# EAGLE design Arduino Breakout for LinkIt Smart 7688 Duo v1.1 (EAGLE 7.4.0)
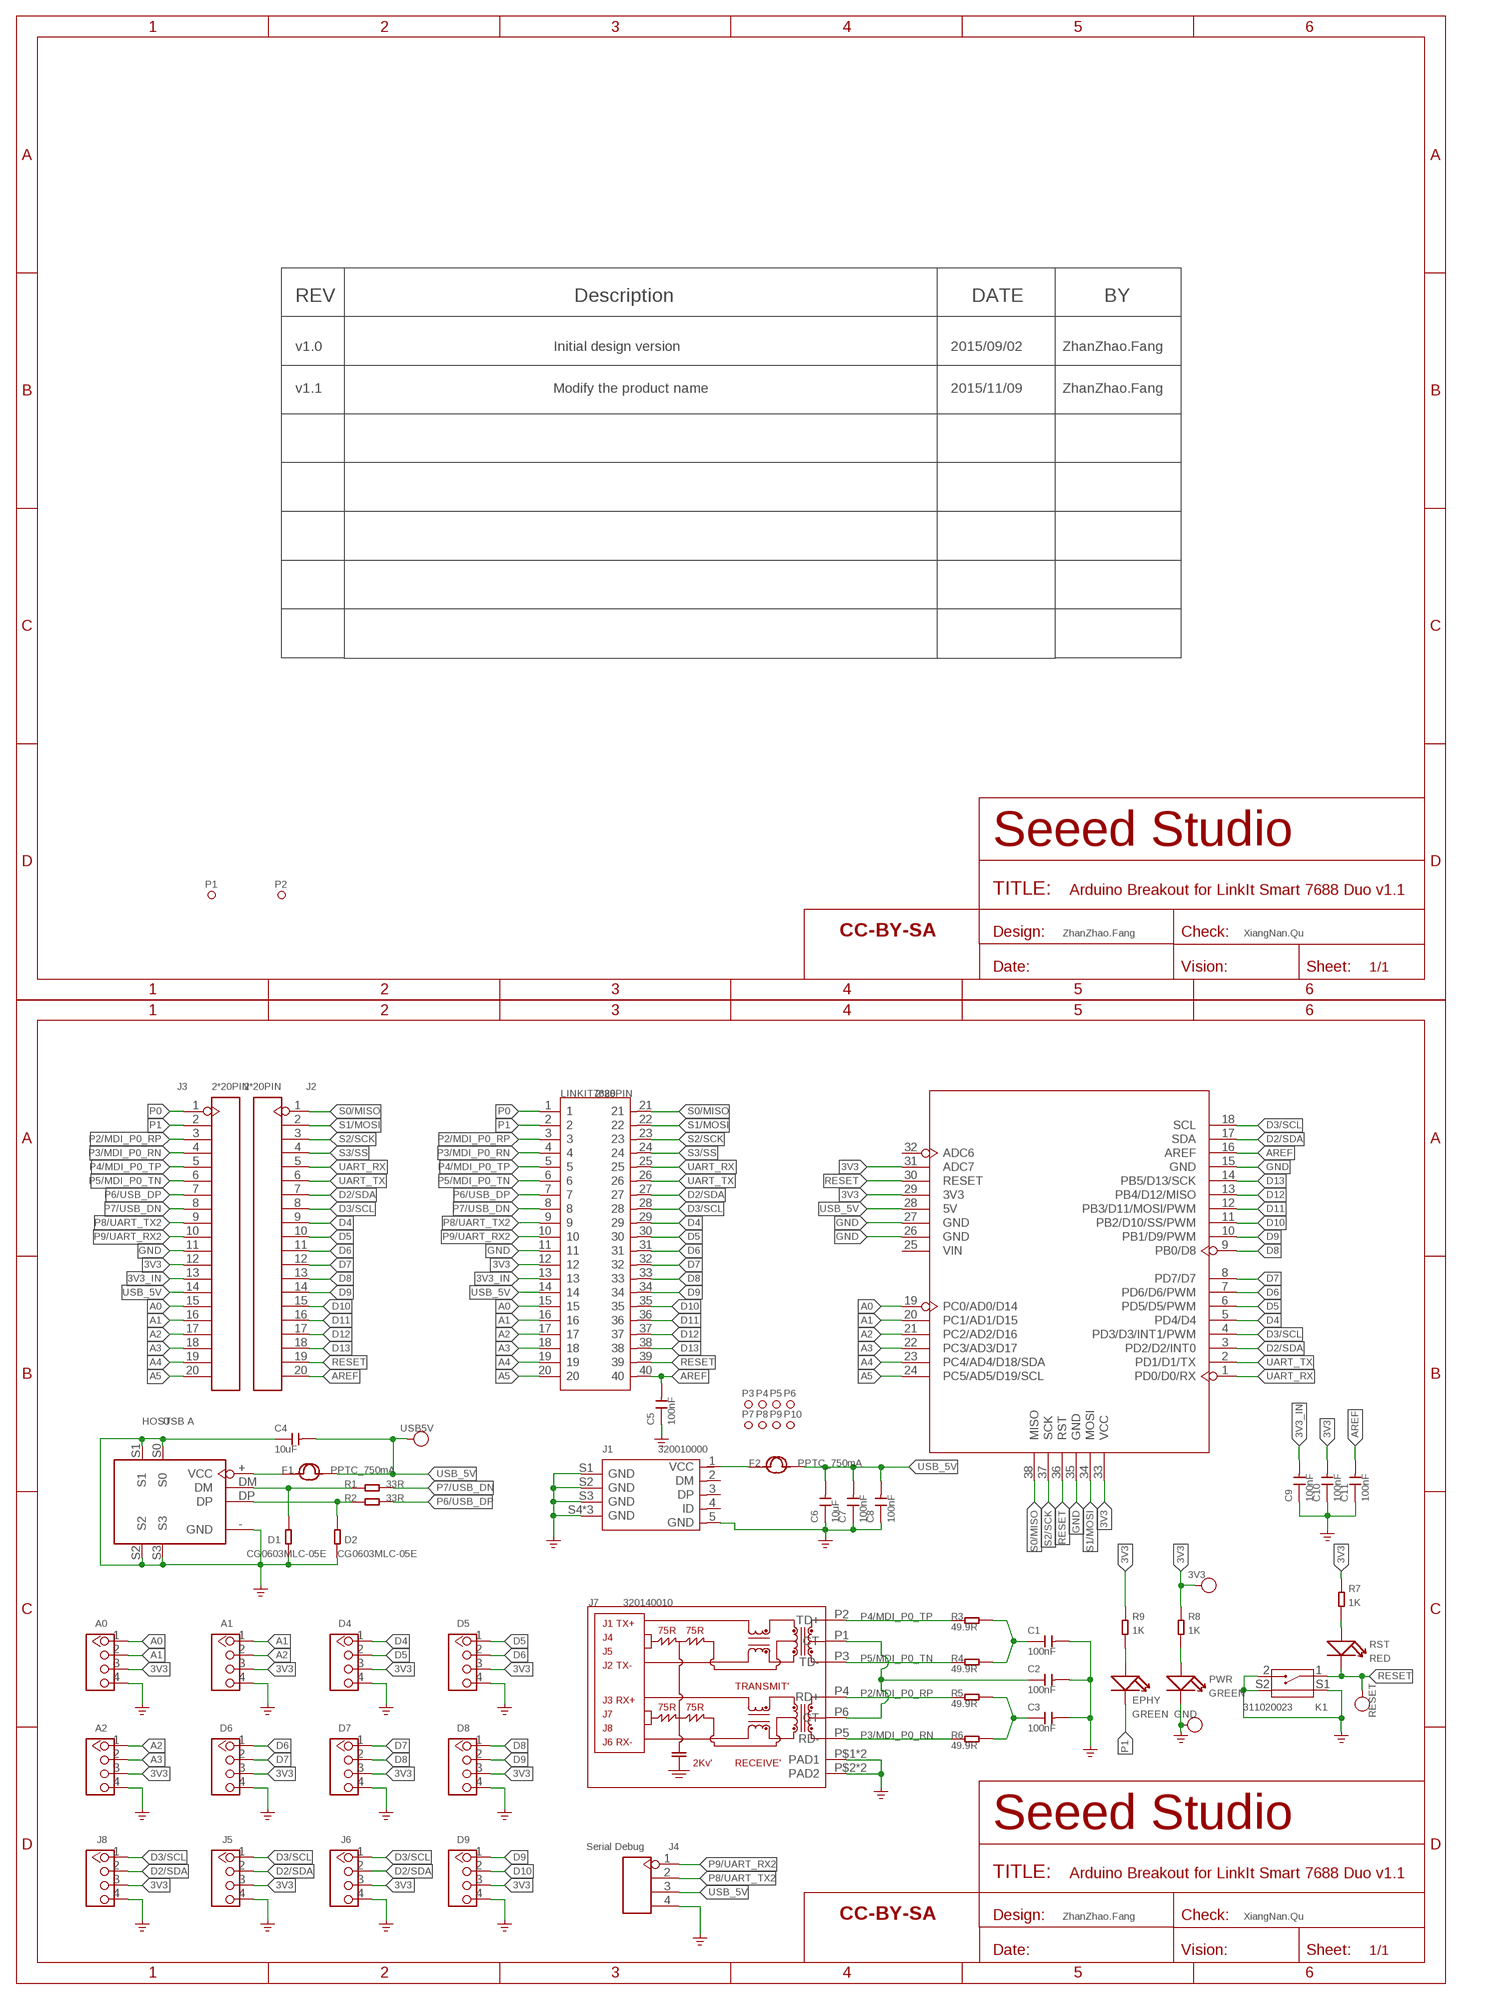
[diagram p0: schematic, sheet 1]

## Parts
3V3  DNP  TEST-POINT'4545'  [TP-D45MIL]
A0  320110033  GROVE-CONNECTOR-DIP-2.0  [HW4-2.0]
A1  320110033  GROVE-CONNECTOR-DIP-2.0  [HW4-2.0]
A2  320110033  GROVE-CONNECTOR-DIP-2.0  [HW4-2.0]
C1  100nF  CAP-0603  [C0603]
C2  100nF  CAP-0603  [C0603]
C3  100nF  CAP-0603  [C0603]
C4  10uF  CAP-0805  [C0805]
C5  100nF  CAP-0603  [C0603]
C6  10uF  CAP-0805  [C0805]
C7  100nF  CAP-0603  [C0603]
C8  100nF  CAP-0603  [C0603]
C9  100nF  CAP-0603  [C0603]
C10  100nF  CAP-0603  [C0603]
C11  100nF  CAP-0603  [C0603]
D1  CG0603MLC-05E  RES-0603  [R0603]
D2  CG0603MLC-05E  RES-0603  [R0603]
D4  320110033  GROVE-CONNECTOR-DIP-2.0  [HW4-2.0]
D5  320110033  GROVE-CONNECTOR-DIP-2.0  [HW4-2.0]
D6  320110033  GROVE-CONNECTOR-DIP-2.0  [HW4-2.0]
D7  320110033  GROVE-CONNECTOR-DIP-2.0  [HW4-2.0]
D8  320110033  GROVE-CONNECTOR-DIP-2.0  [HW4-2.0]
D9  320110033  GROVE-CONNECTOR-DIP-2.0  [HW4-2.0]
EPHY  GREEN  LED'0603'  [LED-0603]
F1  PPTC_750mA  FUSE'1206'  [F1206]
F2  PPTC_750mA  FUSE'1206'  [F1206]
FR1  DNP  SEEEDSTUDIO-OPEN-SCH-FRAME  [SEEEDSTUDIO-PCB-FRAME]
FR2  DNP  SEEEDSTUDIO-OPEN-SCH-FRAME  [SEEEDSTUDIO-PCB-FRAME]
GND  DNP  TEST-POINT'4545'  [TP-D45MIL]
HOST  USB A  USB4+4P-13.2X14.5  [USB4+4-90D-IN]
J1  320010000  MICRO-USB5+4P'5+4P'  [MICRO-USB5+4P-SMD-0.65-B]
J2  2*20PIN  HEADER-20P-2.54  [H20-2.54]
J3  2*20PIN  HEADER-20P-2.54  [H20-2.54]
J4  Serial Debug  HEADER-4P-90D  [H4-2.54-90D-MALE]
J5  320110033  GROVE-CONNECTOR-DIP-2.0  [HW4-2.0]
J6  320110033  GROVE-CONNECTOR-DIP-2.0  [HW4-2.0]
J7  320140010  RJ45-MJ6-BX11-RVS1T073  [RJ45-MJ6-BX11-RVS1T073]
J8  320110033  GROVE-CONNECTOR-DIP-2.0  [HW4-2.0]
K1  311020023  BUTTON-2+2P'TS-1188E'  [SW4-SMD-7.0X3.5X3.5MM-90D]
LINKIT7688  2*20PIN  LINKIT-7688-DUO  [HEADER-2X20P-2.54-65/35MIL]
P1  DNP  MARK-1.0'ANNULAR'  [ROUND-MARK-1.0]
P2  DNP  MARK-1.0'ANNULAR'  [ROUND-MARK-1.0]
P3  MARK-1.0'ANNULAR'  [ROUND-MARK-1.0]
P4  MARK-1.0'ANNULAR'  [ROUND-MARK-1.0]
P5  MARK-1.0'ANNULAR'  [ROUND-MARK-1.0]
P6  MARK-1.0'ANNULAR'  [ROUND-MARK-1.0]
P7  MARK-1.0'ANNULAR'  [ROUND-MARK-1.0]
P8  MARK-1.0'ANNULAR'  [ROUND-MARK-1.0]
P9  MARK-1.0'ANNULAR'  [ROUND-MARK-1.0]
P10  MARK-1.0'ANNULAR'  [ROUND-MARK-1.0]
PWR  GREEN  LED'0603'  [LED-0603]
R1  33R  RES-0603  [R0603]
R2  33R  RES-0603  [R0603]
R3  49.9R  RES-0603  [R0603]
R4  49.9R  RES-0603  [R0603]
R5  49.9R  RES-0603  [R0603]
R6  49.9R  RES-0603  [R0603]
R7  1K  RES-0603  [R0603]
R8  1K  RES-0603  [R0603]
R9  1K  RES-0603  [R0603]
RESET  DNP  TEST-POINT'4545'  [TP-D45MIL]
RST  RED  LED'0603'  [LED-0603]
U2  Shield  ARDUINO-38PWITH-SILK  [ARDUINO-DIM-WITH-SILK]
USB5V  DNP  TEST-POINT'4545'  [TP-D45MIL]

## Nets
3V3: 3V3.T A0.3 A1.3 A2.3 C10.2 D4.3 D5.3 D6.3 D7.3 D8.3 D9.3 J3.12 J5.3 J6.3 J8.3 LINKIT7688.12 R7.2 R8.2 R9.2 U2.29(3V3) U2.31(ADC7) U2.33(VCC)
3V3_IN: C9.2 J3.13 LINKIT7688.13
A0: A0.1 J3.15 LINKIT7688.15 U2.19(PC0/AD0/D14)
A1: A0.2 A1.1 J3.16 LINKIT7688.16 U2.20(PC1/AD1/D15)
A2: A1.2 A2.1 J3.17 LINKIT7688.17 U2.21(PC2/AD2/D16)
A3: A2.2 J3.18 LINKIT7688.18 U2.22(PC3/AD3/D17)
A4: J3.19 LINKIT7688.19 U2.23(PC4/AD4/D18/SDA)
A5: J3.20 LINKIT7688.20 U2.24(PC5/AD5/D19/SCL)
AREF: C5.2 C11.2 J2.20 LINKIT7688.40 U2.16(AREF)
D2/SDA: J2.7 J5.2 J6.2 J8.2 LINKIT7688.27 U2.3(PD2/D2/INT0) U2.17(SDA)
D3/SCL: J2.8 J5.1 J6.1 J8.1 LINKIT7688.28 U2.4(PD3/D3/INT1/PWM) U2.18(SCL)
D4: D4.1 J2.9 LINKIT7688.29 U2.5(PD4/D4)
D5: D4.2 D5.1 J2.10 LINKIT7688.30 U2.6(PD5/D5/PWM)
D6: D5.2 D6.1 J2.11 LINKIT7688.31 U2.7(PD6/D6/PWM)
D7: D6.2 D7.1 J2.12 LINKIT7688.32 U2.8(PD7/D7)
D8: D7.2 D8.1 J2.13 LINKIT7688.33 U2.9(PB0/D8)
D9: D8.2 D9.1 J2.14 LINKIT7688.34 U2.10(PB1/D9/PWM)
D10: D9.2 J2.15 LINKIT7688.35 U2.11(PB2/D10/SS/PWM)
D11: J2.16 LINKIT7688.36 U2.12(PB3/D11/MOSI/PWM)
D12: J2.17 LINKIT7688.37 U2.13(PB4/D12/MISO)
D13: J2.18 LINKIT7688.38 U2.14(PB5/D13/SCK)
GND: A0.4 A1.4 A2.4 C1.2 C2.2 C3.2 C4.1 C5.1 C6.1 C7.1 C8.1 C9.1 C10.1 C11.1 D1.1 D2.1 D4.4 D5.4 D6.4 D7.4 D8.4 D9.4 GND.T HOST.-(GND) HOST.S0 HOST.S1 HOST.S2 HOST.S3 J1.5(GND) J1.S1(GND) J1.S2(GND) J1.S3(GND) J1.S4(GND) J1.S5(GND) J1.S6(GND) J3.11 J4.4 J5.4 J6.4 J7.P$1(PAD1) J7.P$2(PAD2) J7.PAD1 J7.PAD2 J8.4 K1.2 K1.S1 K1.S2 LINKIT7688.11 PWR.- U2.15(GND) U2.26(GND) U2.27(GND) U2.35(GND) ; supply symbol labelled GND_POWER
N$1: PWR.+ R8.1
N$2: EPHY.+ R9.1
N$3: D2.2 HOST.DP R2.1
N$4: D1.2 HOST.DM R1.1
N$5: F1.1 HOST.+(VCC)
N$6: C2.1 J7.P1(CT) J7.P6(CT)
N$7: R7.1 RST.+
N$8: F2.1 J1.1(VCC)
N$10: C1.1 R3.2 R4.2
N$12: C3.1 R5.2 R6.2
P0: J3.1 LINKIT7688.1
P1: EPHY.- J3.2 LINKIT7688.2
P2/MDI_P0_RP: J3.3 J7.P4(RD+) LINKIT7688.3 R5.1
P3/MDI_P0_RN: J3.4 J7.P5(RD-) LINKIT7688.4 R6.1
P4/MDI_P0_TP: J3.5 J7.P2(TD+) LINKIT7688.5 R3.1
P5/MDI_P0_TN: J3.6 J7.P3(TD-) LINKIT7688.6 R4.1
P6/USB_DP: J3.7 LINKIT7688.7 R2.2
P7/USB_DN: J3.8 LINKIT7688.8 R1.2
P8/UART_TX2: J3.9 J4.2 LINKIT7688.9
P9/UART_RX2: J3.10 J4.1 LINKIT7688.10
RESET: J2.19 K1.1 LINKIT7688.39 RESET.T RST.- U2.30(RESET) U2.36(RST)
S0/MISO: J2.1 LINKIT7688.21 U2.38(MISO)
S1/MOSI: J2.2 LINKIT7688.22 U2.34(MOSI)
S2/SCK: J2.3 LINKIT7688.23 U2.37(SCK)
S3/SS: J2.4 LINKIT7688.24
UART_RX: J2.5 LINKIT7688.25 U2.1(PD0/D0/RX)
UART_TX: J2.6 LINKIT7688.26 U2.2(PD1/D1/TX)
USB_5V: C4.2 C6.2 C7.2 C8.2 F1.2 F2.2 J3.14 J4.3 LINKIT7688.14 U2.28(5V) USB5V.T
Unconnected: J1.2(DM) J1.3(DP) J1.4(ID) U2.25(VIN) U2.32(ADC6)

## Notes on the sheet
- REV | Description | DATE | BY
- v1.0 | Initial design version | 2015/09/02 | ZhanZhao.Fang
- v1.1 | Modify the product name | 2015/11/09 | ZhanZhao.Fang
- ZhanZhao.Fang | XiangNan.Qu
- ZhanZhao.Fang | XiangNan.Qu

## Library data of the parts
3V3 GND RESET USB5V = Discrete-new:TEST-POINT; PARTNO: DNP
A0 A1 A2 D4-D9 J5 J6 J8 = Connector-new:GROVE-CONNECTOR-DIP: 4P-2.0:320110033;4P-2.0-90D:320110034
C1-C11 = Discrete-new:CAP: Ceramic Capacitors
D1 D2 R1-R9 = Discrete-new:RES
EPHY PWR RST = Discrete-new:LED
F1 F2 = Discrete-new:FUSE
FR1 FR2 = moudle-new:SEEEDSTUDIO-OPEN-SCH-FRAME
HOST = Connector-new:USB4+4P: 320010017 USB-A-FEMALE
J1 = Connector-new:MICRO-USB5+4P: 5+4P-SMD-0.65-B:320010000;5+2P-SMD-0.65-AB:340032001
J2 J3 = Connector-new:HEADER-20P
J4 = Connector-new:HEADER-4P
J7 = Connector-new:RJ45-MJ6-BX11-RVS1T073: 320140010
K1 = Discrete-new:BUTTON-2+2P: SW4-SMD-4.5X3.8X1.8MM-90D:311020035;SW4-SMD-7.0X3.5X3.5MM-90D:311020023
LINKIT7688 = template:LINKIT-7688-DUO
P1-P10 = Discrete-new:MARK-1.0; PARTNO: DNP
U2 = moudle-new:ARDUINO-38P

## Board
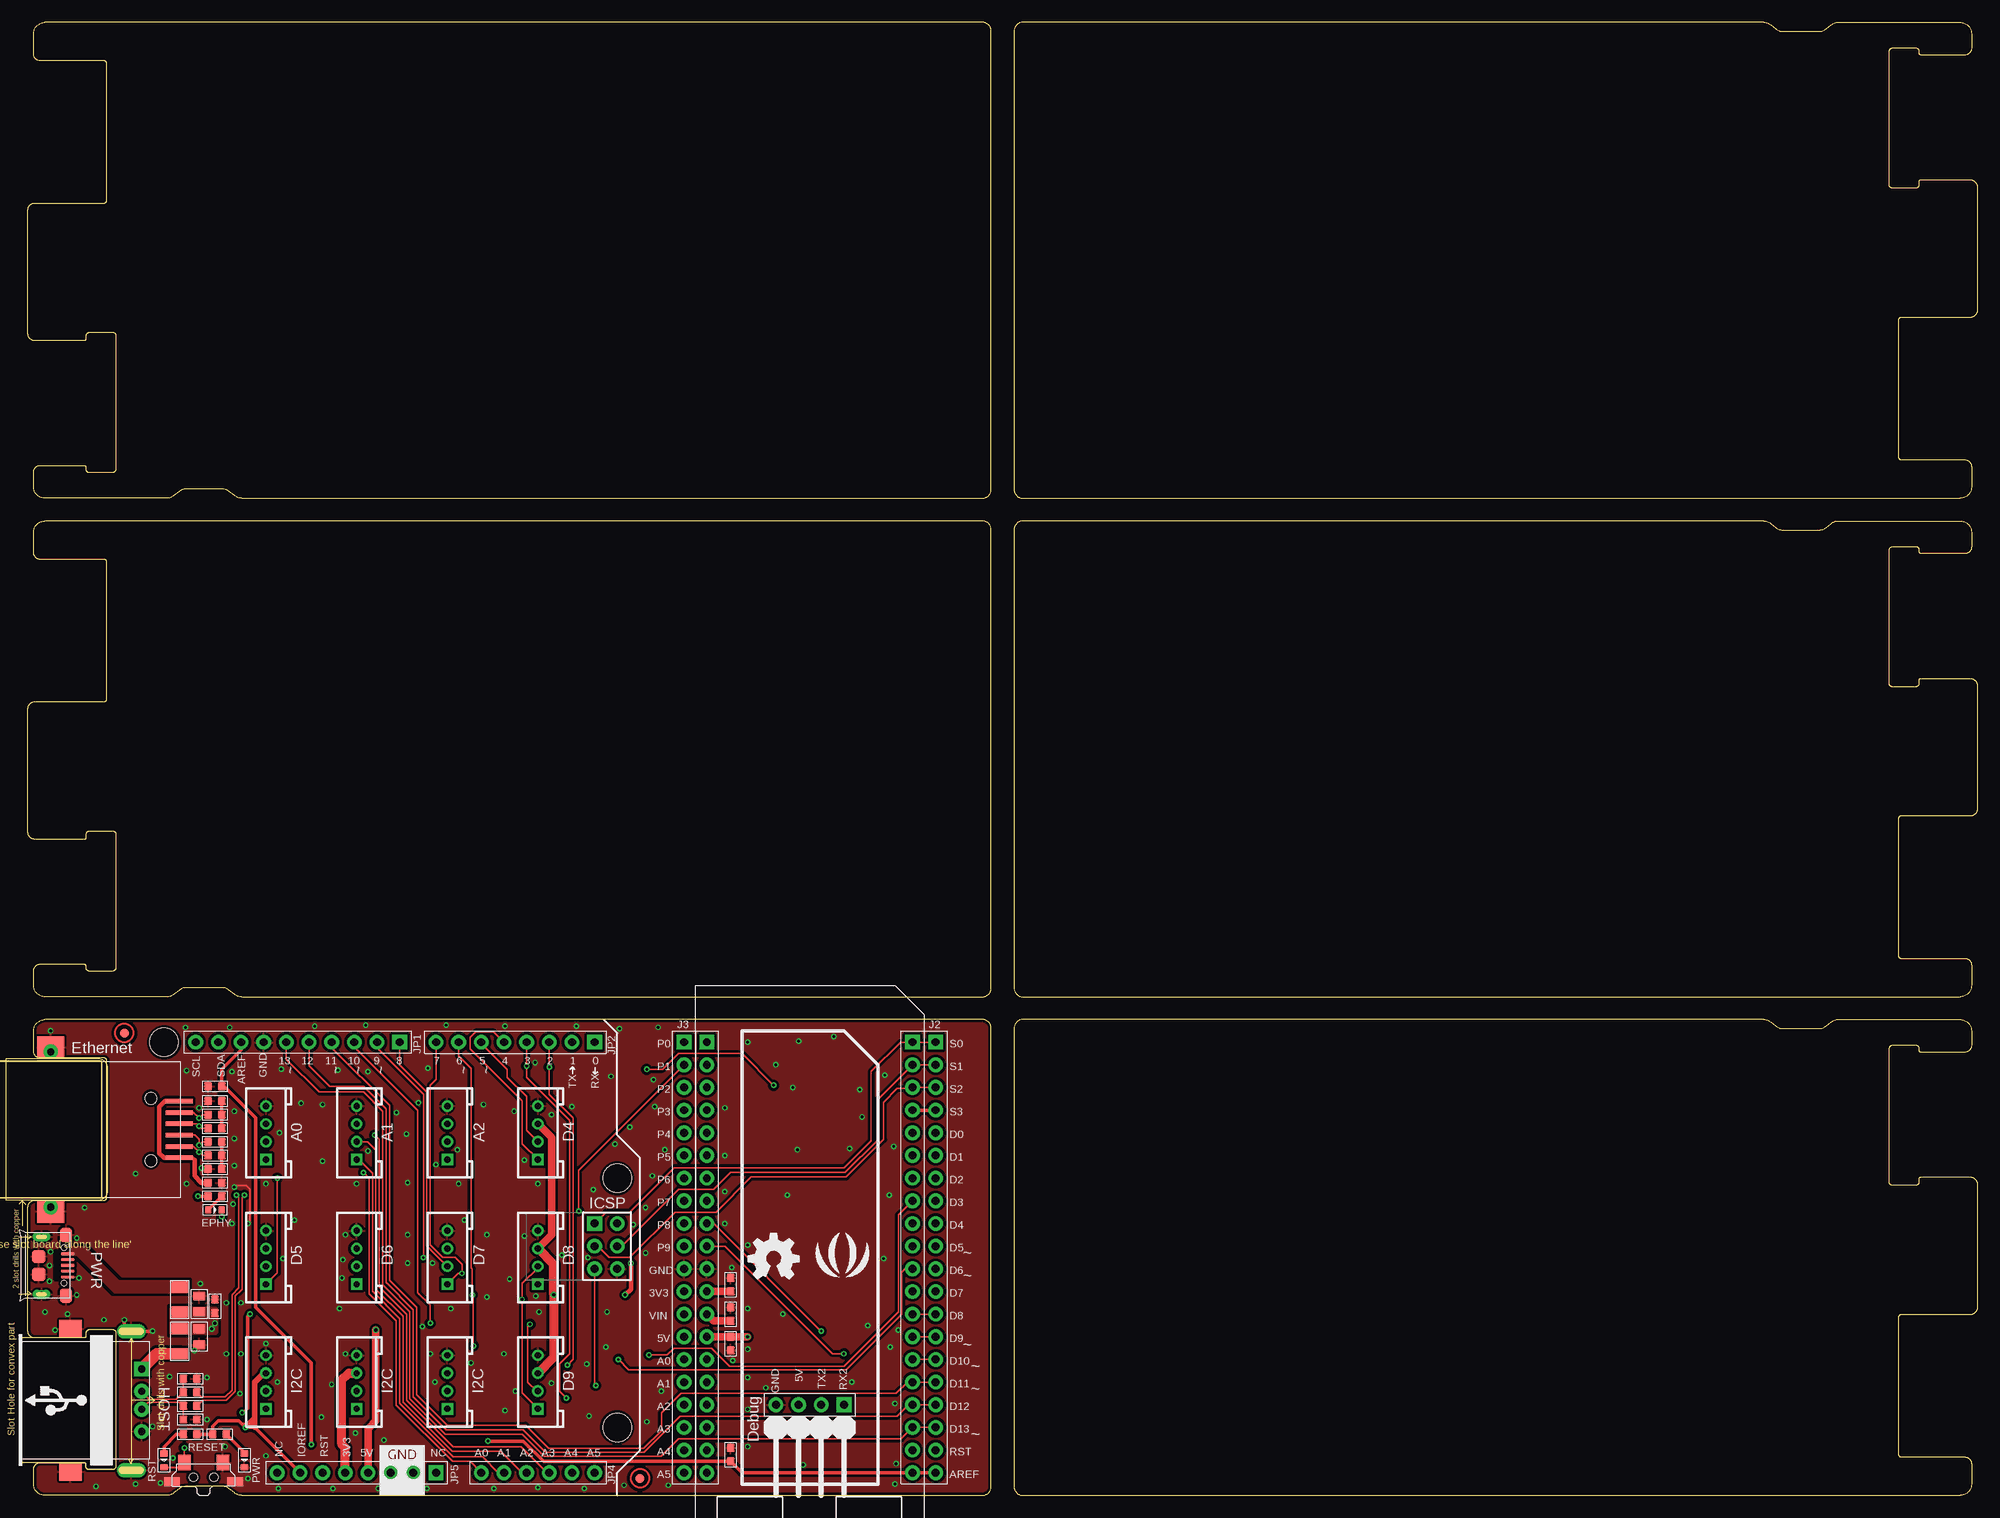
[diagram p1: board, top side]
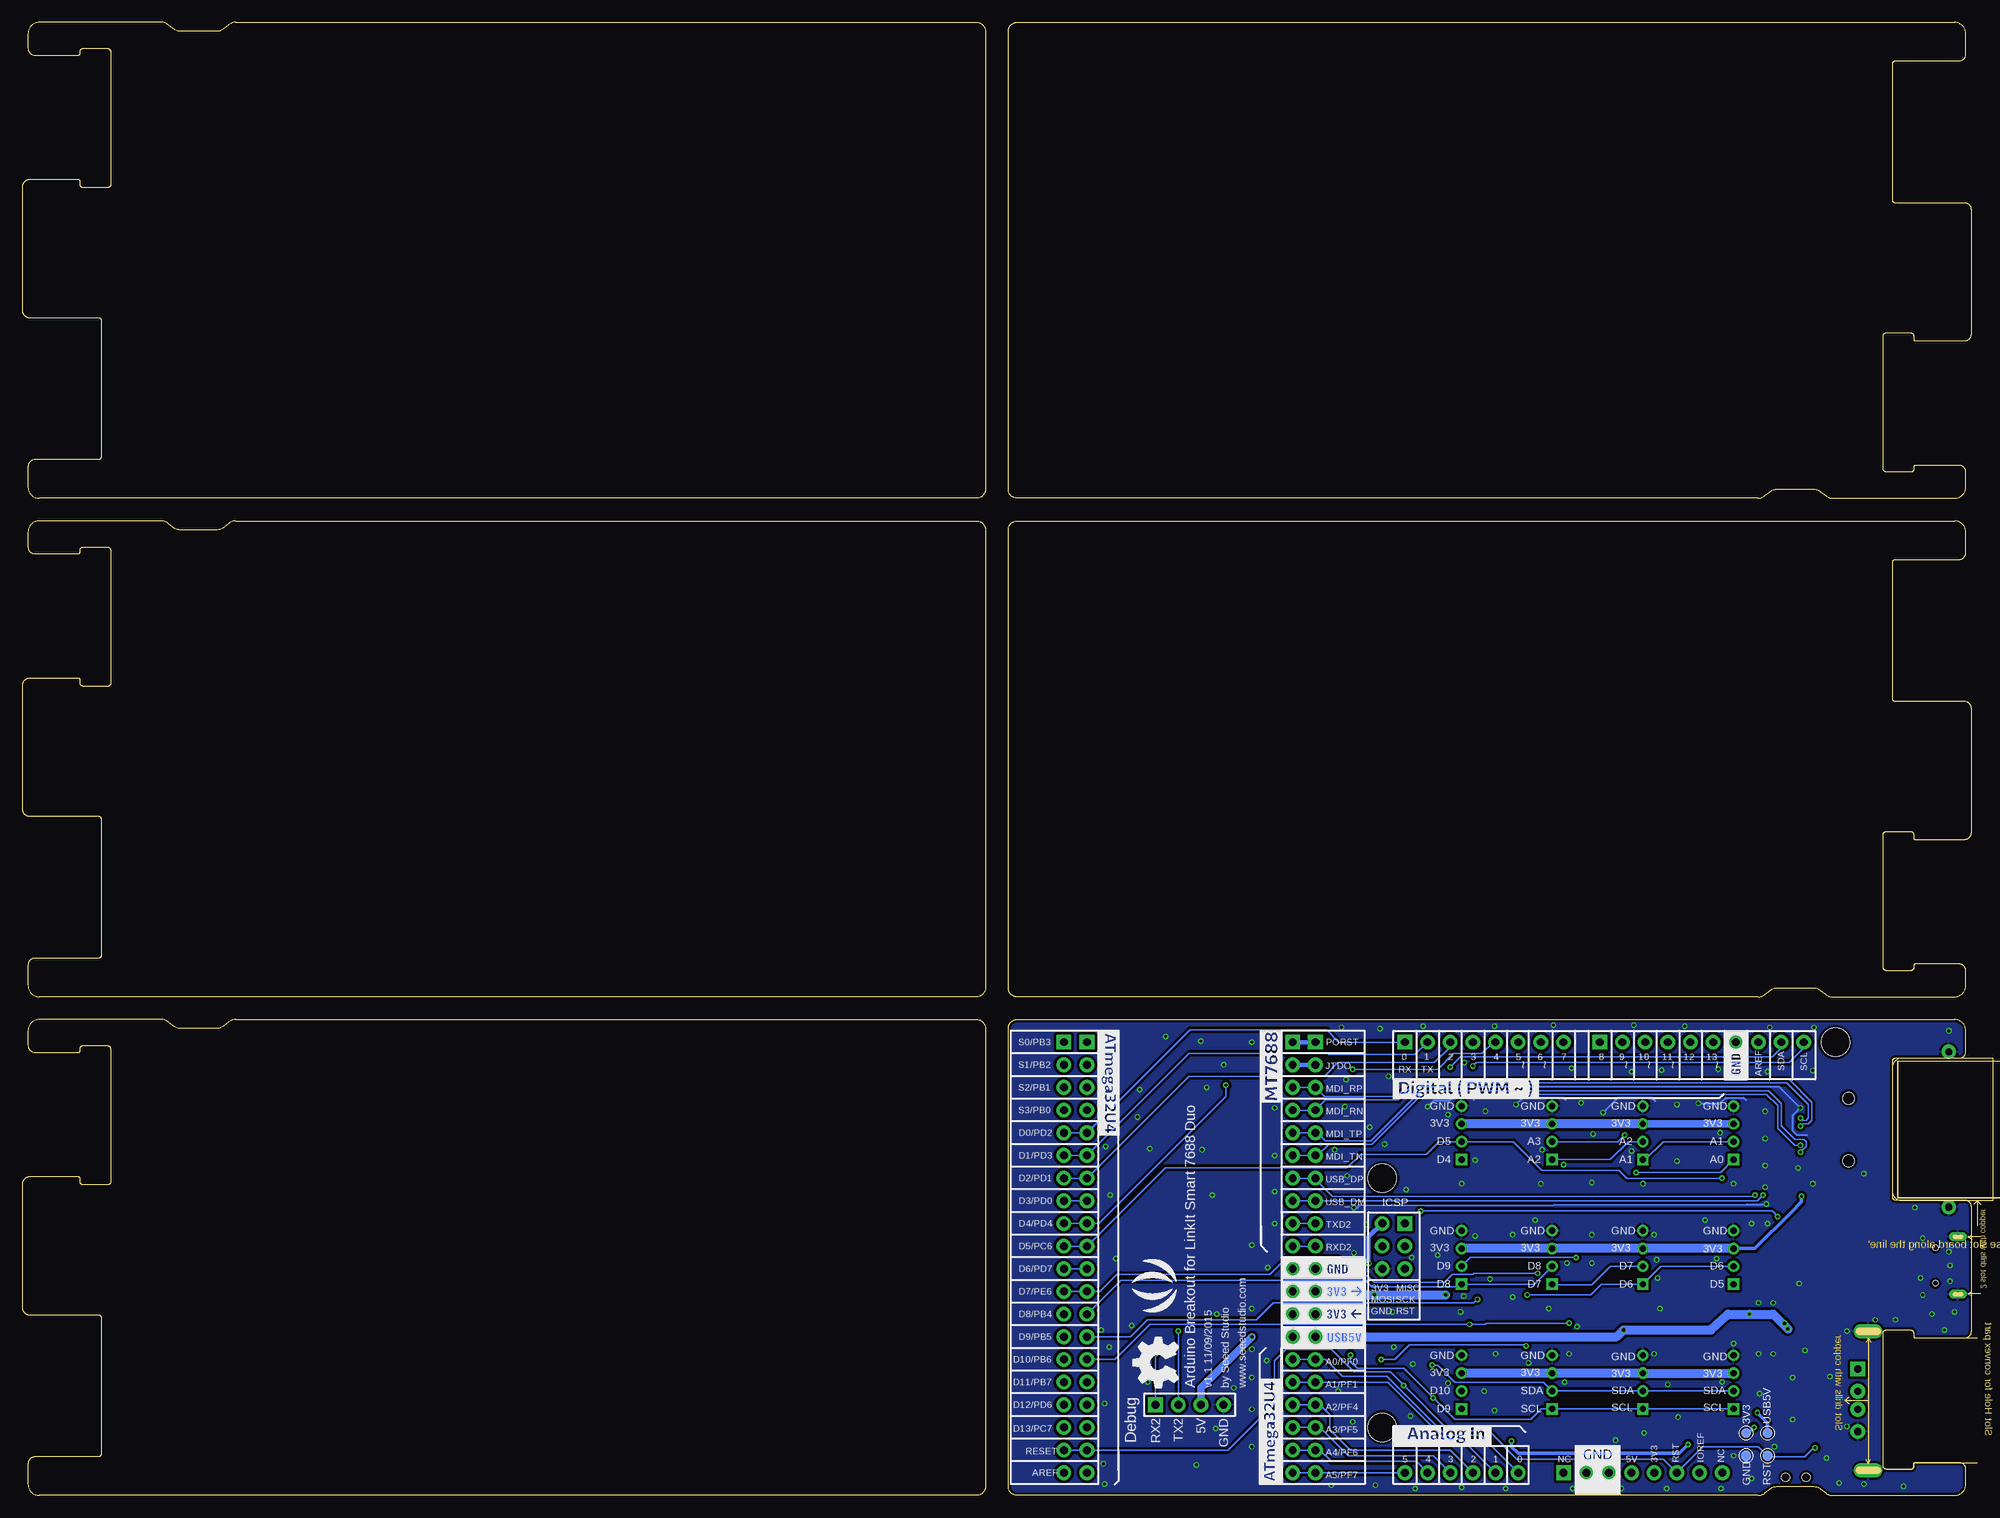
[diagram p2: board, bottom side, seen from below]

Size 219.07 x 165.1 mm. Coordinates in mm from the lower left corner, seen from the top.
Outline: 240 segments
Copper layers (1*16): Top 0.035mm / dielectric 1.5mm / Bottom 0.035mm
Design rules "SeeedStudio_2layer_DRU_no_angle_20140221 *": minimum track width 1mil, minimum drill 12mil, track to track 6mil, track to pad 6mil, pad to pad 6mil, via to via 6mil, smd to smd 0mil, copper to edge 10mil, drill to drill 10mil, minimum pad ring 10mil, minimum via ring 6mil, stop-mask expansion 2mil, vias tented up to drill 25mil, thermal gap 10mil
Holes 2 mm at 3.17,169.54 216.53,169.54 3.17,-4.45 216.53,-4.45

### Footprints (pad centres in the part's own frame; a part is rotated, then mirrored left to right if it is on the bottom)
TP-D45MIL = smd 1.143 x 1.143: T 0,0
HW4-2.0 = drill 0.7 pad 1.27 square: 1 -3,0 | drill 0.7 pad 1.27: 2 -1,0; 3 1,0; 4 3,0
C0603 = smd 0.889 x 0.889: 1 0,0.762; 2 0,-0.762
C0805 = smd 1.397 x 1.016: 1 0,0.889; 2 0,-0.889
R0603 = smd 0.889 x 0.889: 1 0,0.762; 2 0,-0.762
LED-0603 = smd 0.762 x 0.889: + -0.762,0; - 0.762,0
F1206 = smd 1.27 x 1.778: 1 -1.397,0; 2 1.397,0
USB4+4-90D-IN = drill 0.813 pad 1.651 square: + 0.85,-3.5 | drill 0.813 pad 1.651: - 0.85,3.5; DM 0.85,-1; DP 0.85,1 | smd 2.54 x 2.032: S0 8.83,8.001; S3 8.83,-8.001 | drill 0.7 pad 1.6 long: S1 2,7.874; S2 2,-7.747
MICRO-USB5+4P-SMD-0.65-B = smd 0.381 x 1.524: 1 -1.3,-0.25; 2 -0.65,-0.25; 3 0,-0.25; 4 0.65,-0.25; 5 1.3,-0.25 | smd 1.6 x 1.397: S1 -3.4,-0.427; S6 3.4,-0.427 | drill 0.508 pad 1.016 long: S2 -3.226,-3.175; S5 3.226,-3.175 | smd 1.5 x 1.5: S3 -1,-3.5; S4 1,-3.5 | hole 0.635: -2,-0.65; 2,-0.65
H20-2.54 = drill 0.889 pad 1.651 square: 1 0,-24.13 | drill 0.889 pad 1.651: 2 0,-21.59; 3 0,-19.05; 4 0,-16.51; 5 0,-13.97; 6 0,-11.43; 7 0,-8.89; 8 0,-6.35; 9 0,-3.81; 10 0,-1.27; 11 0,1.27; 12 0,3.81; 13 0,6.35; 14 0,8.89; 15 0,11.43; 16 0,13.97; 17 0,16.51; 18 0,19.05; 19 0,21.59; 20 0,24.13
H4-2.54-90D-MALE = drill 0.889 pad 1.651 square: 1 0,3.81 | drill 0.889 pad 1.651: 2 0,1.27; 3 0,-1.27; 4 0,-3.81
RJ45-MJ6-BX11-RVS1T073 = smd 0.5 x 3: P1 3.175,14.4; P2 1.905,14.4; P3 0.635,14.4; P4 -0.635,14.4; P5 -1.905,14.4; P6 -3.175,14.4 | smd 2.5 x 3: P$1 -9.2,0; P$2 9.2,0 | drill 0.8 pad 1.6: PAD1 -8.7,0; PAD2 8.7,0 | hole 1.35: -3.5,11.24; 3.5,11.24
SW4-SMD-7.0X3.5X3.5MM-90D = smd 1.397 x 1.778: 1 -2.159,1.651; 2 2.159,1.651 | smd 1.778 x 1.016: S1 -3.556,-0.508; S2 3.556,-0.508 | hole 0.95: -1.15,0; 1.15,0
HEADER-2X20P-2.54-65/35MIL = drill 0.889 pad 1.651 square: 1 0,24.13; 21 23.05,24.13 | drill 0.889 pad 1.651: 2 0,21.59; 3 0,19.05; 4 0,16.51; 5 0,13.97; 6 0,11.43; 7 0,8.89; 8 0,6.35; 9 0,3.81; 10 0,1.27; 11 0,-1.27; 12 0,-3.81; 13 0,-6.35; 14 0,-8.89; 15 0,-11.43; 16 0,-13.97; 17 0,-16.51; 18 0,-19.05; 19 0,-21.59; 20 0,-24.13; 22 23.05,21.59; 23 23.05,19.05; 24 23.05,16.51; 25 23.05,13.97; 26 23.05,11.43; 27 23.05,8.89; 28 23.05,6.35; 29 23.05,3.81; 30 23.05,1.27; 31 23.05,-1.27; 32 23.05,-3.81; 33 23.05,-6.35; 34 23.05,-8.89; 35 23.05,-11.43; 36 23.05,-13.97; 37 23.05,-16.51; 38 23.05,-19.05; 39 23.05,-21.59; 40 23.05,-24.13
ROUND-MARK-1.0 = smd 1.016 x 1.016: P$1 0,0
ARDUINO-DIM-WITH-SILK = drill 0.889 pad 1.651 square: 1 63.5,50.8; 9 41.656,50.8; 25 45.72,2.54; 38 63.5,30.48 | drill 0.889 pad 1.651: 2 60.96,50.8; 3 58.42,50.8; 4 55.88,50.8; 5 53.34,50.8; 6 50.8,50.8; 7 48.26,50.8; 8 45.72,50.8; 10 39.116,50.8; 11 36.576,50.8; 12 34.036,50.8; 13 31.496,50.8; 14 28.956,50.8; 15 26.416,50.8; 16 23.876,50.8; 17 21.336,50.8; 18 18.796,50.8; 19 50.8,2.54; 20 53.34,2.54; 21 55.88,2.54; 22 58.42,2.54; 23 60.96,2.54; 24 63.5,2.54; 26 43.18,2.54; 27 40.64,2.54; 28 38.1,2.54; 29 35.56,2.54; 30 33.02,2.54; 31 30.48,2.54; 32 27.94,2.54; 33 66.04,30.48; 34 66.04,27.94; 35 66.04,25.4; 36 63.5,25.4; 37 63.5,27.94 | hole 3.2: 15.24,50.8; 66.04,35.56; 66.04,7.62

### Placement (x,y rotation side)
3V3  25.91,6.99 0 bottom
A0  27.3,40.64 90 top
A1  37.46,40.64 90 top
A2  47.62,40.64 90 top
C1  21.59,36.58 270 top
C2  21.59,35.05 90 top
C3  21.59,44.2 270 top
C4  19.81,17.78 180 top
C5  21.59,45.85 90 top
C6  19.81,21.46 0 top
C7  21.59,21.21 0 top
C8  79.38,17.02 180 top
C9  79.38,20.32 0 top
C10  79.38,23.62 0 top
C11  79.38,4.57 0 top
D1  18.8,13.08 270 top
D2  18.8,8.51 270 top
D4  57.78,40.64 90 top
D5  27.3,26.67 90 top
D6  37.46,26.67 90 top
D7  47.62,26.67 90 top
D8  57.78,26.67 90 top
D9  57.78,12.7 90 top
EPHY  21.59,32 0 top
F1  17.65,17.27 90 top
F2  17.65,21.97 270 top
FR1  not placed on the board
FR2  not placed on the board
GND  25.91,4.45 0 bottom
HOST  14.22,10.67 180 top
J1  5.33,25.78 270 top
J2  102.36,26.67 180 top
J3  74.17,26.67 180 top
J4  88.27,10.16 270 top
J5  37.46,12.7 90 top
J6  47.62,12.7 90 top
J7  3.17,41.02 270 top
J8  27.3,12.7 90 top
K1  20.32,2.03 0 top
LINKIT7688  76.71,26.67 0 top
P1  69.22,1.91 0 top
P2  11.43,51.82 0 top
P3  not placed on the board
P4  not placed on the board
P5  not placed on the board
P6  not placed on the board
P7  not placed on the board
P8  not placed on the board
P9  not placed on the board
P10  not placed on the board
PWR  24.89,3.94 270 top
R1  18.8,11.56 90 top
R2  18.8,10.03 90 top
R3  21.59,38.1 90 top
R4  21.59,39.62 90 top
R5  21.59,41.15 90 top
R6  21.59,42.67 90 top
R7  18.8,6.86 90 top
R8  22.1,6.86 270 top
R9  21.59,33.53 270 top
RESET  23.49,4.45 0 bottom
RST  15.88,3.94 270 top
U2  0.63,0 0 top
U$20  [OSHW_FILLX200_NOTEXT]  89.54,12.06 90 bottom
U$21  [SEEED-SILK-280*268MIL]  91.44,23.5 90 bottom
U$22  [OSHW_FILLX200_NOTEXT]  81.36,24.28 0 top
U$23  [SEEED-SILK-280*268MIL]  91.9,26.16 0 top
USB5V  23.49,6.99 0 bottom

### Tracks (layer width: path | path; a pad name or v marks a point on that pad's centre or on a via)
3V3  (via drill 0.3, 0.36, 0.38)
  Top 0.406: 24.64,8 24.26,8.38 21.97,8.38 21.34,7.75 R8.2 R7.2 | 24.64,8 v25.02,7.62 26.03,7.62 U2.31 | 24.64,8 25.53,8 | R9.2 v19.69,33.53
  Top 0.508: v67.56,22.48 68.2,23.11 v68.2,26
  Top 0.61: J8.3 27.03,13.7 26.03,12.7 26.03,8.64 | 26.03,8.64 25.65,8.26 | 25.65,8.26 v25.02,7.62 | 25.65,8.26 25.65,7.75 | 26.03,7.62 26.03,8.64
  Top 0.813: D4.3 59.31,40.12 59.31,29.19 D8.3 | C10.2 LINKIT7688.12
  Top 1.016: U2.29 36.2,5.33 35.81,5.71 35.81,12.94 36.58,13.7 J5.3 | D8.3 59.56,25.89 v59.56,22.48 59.56,15.48 D9.3
  Bottom 0.406: 3V3.T 25.65,6.99 v25.02,7.62 | D5.3 24.91,27.67 20.89,31.69 20.83,31.75 19.69,32.89 v19.69,33.53
  Bottom 0.508: U2.33 68.2,28.96 v68.2,26
  Bottom 0.813: A0.3 A1.3
  Bottom 1.016: D9.3 J6.3 J5.3 J8.3 | LINKIT7688.12 J3.12 69.09,22.86 68.71,22.48 v67.56,22.48 v59.56,22.48 | D5.3 D6.3 D7.3 D8.3 | A1.3 A2.3 D4.3
3V3_IN
  Top 0.813: C9.2 77.47,19.56 LINKIT7688.13
  Bottom 0.813: J3.13 LINKIT7688.13
A0  (via drill 0.3)
  Top 0.152: U2.19 50.16,3.81 48.23,3.81 41.91,10.13 41.91,19.56 38.86,22.61 38.86,35.56 v38.23,36.2
  Bottom 0.152: LINKIT7688.15 J3.15 73.03,15.24 71.12,13.34 66.17,13.34 59.56,6.73 55.63,6.73 U2.19 | v38.23,36.2 28.75,36.2 A0.1
A1
  Top 0.152: U2.20 53.34,2.54 51.56,4.32 48.28,4.32 42.29,10.31 42.29,19.81 39.24,22.86 39.24,36.07 37.67,37.64 A1.1
  Bottom 0.152: LINKIT7688.16 J3.16 66.04,12.7 59.69,6.35 57.78,6.35 U2.20 | A1.1 37.16,37.64 35.18,39.62 27.32,39.62 A0.2
A2
  Top 0.152: U2.21 56.01,2.54 53.59,4.95 48.19,4.95 42.67,10.47 42.67,20.07 39.62,23.11 39.62,38.73 38.72,39.64 A1.2
  Bottom 0.152: LINKIT7688.17 J3.17 73.66,10.16 72.52,9.02 72.52,7.37 70.23,5.08 59.05,5.08 U2.21 | A2.1 41.1,37.64 39.1,39.64 A1.2
A3  (via drill 0.3)
  Top 0.152: U2.22 58.8,2.54 55.88,5.46 48.28,5.46 43.05,10.69 43.05,20.32 40,23.37 40,39.88 v39.5,40.39
  Bottom 0.152: LINKIT7688.18 J3.18 73.66,7.62 70.48,4.45 60.96,4.45 U2.22 | A2.2 40.24,39.64 v39.5,40.39
A4
  Bottom 0.152: LINKIT7688.19 J3.19 73.66,5.08 72.39,3.81 62.86,3.81 U2.23
A5
  Bottom 0.152: LINKIT7688.20 J3.20 U2.24
AREF  (via drill 0.3)
  Top 0.406: U2.16 24.51,49.91 22.35,47.75 C5.2 22.61,45.85 26.16,42.29 26.16,21.08 32.38,14.86 v32.38,5.71 | J2.20 LINKIT7688.40 80.65,2.54 C11.2 58.42,3.81 56.13,6.1 v52.2,6.1
  Bottom 0.406: v52.2,6.1 52.2,5.46 51.43,4.7 33.4,4.7 v32.38,5.71
D2/SDA  (via drill 0.3)
  Top 0.152: U2.3 v59.05,48.01 59.05,44.96 61.72,42.29 61.72,15.24 v61.09,14.61
  Bottom 0.152: J2.7 LINKIT7688.27 88.33,46.99 73.15,46.99 71.63,48.51 60.83,48.51 59.05,50.29 U2.3 | U2.17 21.97,50.16 22.99,49.15 57.91,49.15 v59.05,48.01 | v61.09,14.61 60.45,14.61 58.55,12.7 48.62,12.7 J6.2 J5.2 J8.2
D3/SCL  (via drill 0.3)
  Top 0.152: U2.4 v56.52,48.13 56.52,46.86 61.34,42.04 61.34,15.88 60.2,14.73 60.2,11.68 v60.96,10.92 | LINKIT7688.28 98.17,31.43 98.17,20.57 92.08,14.48 79.25,14.48 77.22,16.51 73.03,16.51 72.26,15.75 v70.23,15.75
  Bottom 0.152: U2.18 19.43,50.16 21.08,48.51 56.13,48.51 v56.52,48.13 | LINKIT7688.28 J2.8 | v70.23,15.75 70.23,14.99 69.47,14.22 64.26,14.22 v60.96,10.92 58.55,8.51 50.04,8.51 48.85,9.7 J6.1 J5.1 J8.1
D4  (via drill 0.3)
  Top 0.152: U2.5 52.83,51.94 50.8,51.94 50.16,51.31 50.16,50.04 56.01,44.2 56.01,39.42 D4.1 | v69.98,47.75 71.76,47.75 73.53,49.53 80.65,49.53 v84.2,45.97
  Bottom 0.152: J2.9 LINKIT7688.29 98.43,30.48 84.2,44.7 v84.2,45.97 | v69.98,47.75 60.45,47.75 58.67,49.53 55.5,49.53 54.23,50.8 U2.5
D5  (via drill 0.3)
  Top 0.152: U2.6 51.43,50.67 54.36,47.75 54.36,46.86 56.52,44.7 56.52,40.91 D4.2 | v28.58,35.56 28.58,24.94 D5.1
  Bottom 0.152: J2.10 LINKIT7688.30 91,36.7 70.61,36.7 69.09,38.23 61.72,38.23 60.32,39.62 57.8,39.62 D4.2 51.96,39.64 48.77,36.45 40.13,36.45 39.24,35.56 v28.58,35.56
D6  (via drill 0.3)
  Top 0.152: U2.7 48.89,49.28 50.29,47.88 50.29,25.53 50.42,25.4 v50.42,22.48 50.55,22.35 v50.55,16.76 | LINKIT7688.31 98.93,25.4 98.55,25.02 98.55,20.32 92.33,14.1 67.95,14.1 v66.8,15.24
  Bottom 0.152: LINKIT7688.31 J2.11 | D5.2 35.46,25.67 D6.1 42.12,23.67 43.31,22.48 v50.42,22.48 | v66.8,15.24 65.28,15.24 63.63,16.89 50.67,16.89 v50.55,16.76
D7  (via drill 0.3)
  Top 0.152: U2.8 46.35,46.61 45.72,45.97 45.72,28.07 47.12,26.67 48.51,26.67 49.28,25.91 v49.28,24.89 48.85,24.89 D7.1
  Bottom 0.152: J2.12 LINKIT7688.32 98.3,22.86 96.39,24.77 79.25,24.77 77.34,26.67 71.63,26.67 69.6,24.64 68.33,24.64 67.56,23.88 59.69,23.88 58.8,24.77 56.52,24.77 56.39,24.89 v49.28,24.89 | D6.2 41.13,25.67 43.18,23.62 47.58,23.62 D7.1
D8
  Top 0.152: J2.13 LINKIT7688.33 | D7.2 45.34,27.96 45.34,45.21 42.29,48.26 U2.9
  Bottom 0.152: LINKIT7688.33 95.95,24.13 68.58,24.13 67.82,23.37 58.09,23.37 D8.1 49.62,23.67 D7.2 47.77,25.53
D9  (via drill 0.3)
  Top 0.152: U2.10 39.75,50.16 44.96,44.96 v44.96,26.67 | J2.14 LINKIT7688.34 | D9.1 56.01,11.48 v56.01,21.97 56.01,23.75 57.78,25.53 D8.2
  Bottom 0.152: v56.01,21.97 56.39,21.59 78.87,21.59 80.77,19.68 92.96,19.68 94.87,17.78 LINKIT7688.34 | v44.96,26.67 56.78,26.67 D8.2
D10  (via drill 0.3)
  Top 0.152: U2.11 37.21,50.29 44.32,43.18 44.32,22.73 45.72,21.34 v45.72,19.3 | LINKIT7688.35 J2.15 | D9.2 57.64,11.7 56.64,12.7 56.64,18.92 v56.9,19.18
  Bottom 0.152: v45.72,19.3 54.99,19.3 55.12,19.18 v56.9,19.18 92.71,19.18 96.65,15.24 LINKIT7688.35
D11
  Top 0.152: J2.16 LINKIT7688.36 99.19,12.7 97.92,11.43 73.81,11.43 71.63,9.24 71.63,7.24 69.65,5.26 59,5.26 56.39,7.87 47.62,7.87 44.2,11.3 44.2,21.08 41.15,24.13 41.15,43.69 34.67,50.16 U2.12
D12
  Top 0.152: U2.13 32.13,48.13 34.42,45.85 38.23,45.85 40.77,43.31 40.77,23.88 43.81,20.83 43.81,11.05 47.5,7.37 56.13,7.37 58.64,4.86 69.7,4.86 73.73,8.89 98.04,8.89 99.31,10.16 LINKIT7688.37 J2.17
D13
  Top 0.152: U2.14 29.59,48.9 33.27,45.21 38.23,45.21 40.39,43.05 40.39,23.62 43.43,20.57 43.43,10.83 47.41,6.86 56.01,6.86 58.47,4.4 71.58,4.4 73.53,6.35 98.49,6.35 LINKIT7688.38 J2.18
GND  (via drill 0.3)
  Top 0.203: v25.27,30.48 25.53,30.73 25.53,34.29 25.15,34.67 23.88,34.67 v23.75,34.54
  Top 0.406: v11.43,19.68 11.43,19.18 12.19,18.41 v14.61,18.41
  Top 0.61: C1.2 20.19,36.58 v20.07,36.7
  Bottom 0.203: v69.85,32.26 69.47,32.26 69.22,32.51 25.78,32.64 v23.62,32.64 | 63.75,44.58 62.55,45.78 22.16,45.78 v19.81,43.43 20.7,42.55 20.7,40.89 20.19,40.39 19.05,40.39 | 56.39,44.32 56.64,44.58 58.8,44.58 59.18,44.2 60.96,44.2 v61.59,43.56 | 46.1,44.32 46.35,44.58 50.93,44.58 v51.69,43.81 | 36.07,44.2 36.45,44.58 40.26,44.58 v41.91,42.93 | v31.24,43.94 28.83,43.94 28.19,44.58 26.16,44.58 25.91,44.32
  other vias: 24.38,11.43 20.7,13.21 19.3,16.26 16.51,13.34 14.61,7.75 16.89,4.19 22.73,5.46 25.27,1.91 27.3,4.45 12.7,1.27 15.49,1.4 8.25,1.02 6.98,32.26 9.14,19.68 23.75,36.96 12.7,36.07 18.41,34.92 18.41,47.62 3.17,52.07 23.49,47.5 29.02,47.78 33.66,43.81 35.36,47.65 38.73,47.5 23.75,43.05 23.75,40.01 28.83,40.64 33.66,37.47 27.3,34.92 37.46,34.92 30.48,30.86 36.2,29.21 35.81,24.38 52.07,22.23 43.18,29.21 43.18,35.05 56.26,29.08 49.53,30.86 48.89,34.92 57.78,34.92 54.61,24.26 44.83,18.92 45.72,15.88 46.23,12.7 53.98,15.88 50.29,14.86 54.1,9.53 40.51,6.19 37.34,6.99 33.53,8.76 28.7,0.76 34.8,0.76 39.88,0.76 45.34,0.76 52.83,0.76 57.78,0.89 62.99,0.76 63.52,8.89 71.63,11.68 69.98,8.26 27.3,17.02 65.41,16.64 69.85,27.18 70.61,35.81 55.12,43.05 59.31,42.67 70.87,43.56 68.07,41.27 64.01,34.29 45.47,47.88 44.38,44 43.05,40.51 52.07,29.21 68.45,30.35 65.98,46.96 70.74,46.61 66.93,52.32 71.25,52.45 62.1,52.58 54.1,52.58 47.5,52.7 38.48,52.7 32.77,52.58 23.24,52.45 18.29,52.45 78.74,43.43 86.87,38.73 78.74,38.1 86.36,45.72 84.45,48.26 81.28,50.8 87,50.93 90.93,51.44 96.65,47.12 93.85,45.47 92.71,38.86 97.66,39.12 94.11,42.42 97.16,33.66 85.73,33.66 78.74,30.48 81.28,28.07 96.52,26.54 94.74,19.05 81.28,20.95 81.28,13.21 85.22,20.32 92.96,12.7 97.28,16.64 98.17,18.54 97.79,10.29 83.31,12.06 81.28,16.38 81.28,9.65 79.63,15.11 85.34,7.49 97.92,3.56 87.5,3.43 81.28,5.46 67.44,1.14 72.39,1.14 97.79,1.27 43.18,26.04 45.97,26.04 57.47,48.53 66.42,39.37 72.01,38.73 36.2,15.88 34.67,12.45 28.58,12.7 38.73,38.61 48.77,38.73 56.26,37.59 35.94,26.42 29.21,26.54 57.53,22.35 55.24,11.68 60.45,26.92 59.31,12.57 63.25,14.73 63.37,26.67 79.5,25.53 24.51,15.88 22.86,15.88 24.51,21.59 22.86,21.59 23.49,30.48 3.05,24 3.05,25.78 3.17,27.3 6.1,28.83 3.68,18.54 5.08,20.32 2.54,20.57 20.7,8.51 19.94,23.75 78.74,34.04 6.1,22.48 6.35,24.38 46.35,37.08 35.56,20.95 48.01,20.95 57.91,20.57 65.53,20.57
  pour Bottom (isolate 0.305, rank 3): 1.52,54.86 108.97,54.86 111.25,52.2 111.25,1.14 109.73,-0.64 1.78,-0.64 0.38,0.76 0.38,53.72
  pour Top (isolate 0.305, rank 3): 1.14,54.36 108.46,54.36 110.87,51.69 110.87,0.64 109.22,-1.14 1.4,-1.14 0,0.25 0,53.21
N$1
  Top 0.406: R8.1 24.89,4.83 PWR.+
N$2
  Top 0.406: R9.1 EPHY.+
N$3
  Top 0.152: HOST.DP 13.37,9.69 14.1,10.41 17.65,10.41 R2.1 D2.2
N$4
  Top 0.152: HOST.DM 13.37,11.64 14.22,10.79 17.27,10.79 R1.1 D1.2
N$5
  Top 1.27: HOST.+ 15.08,15.88 F1.1
N$6
  Top 0.508: J7.P6 16,44.2 15.37,43.56 15.37,38.35 15.88,37.85 J7.P1 19.05,37.85 19.3,37.59 19.3,35.81 20.07,35.05 C2.1
N$7
  Top 0.406: RST.+ 15.88,5.46 17.27,6.86 R7.1
N$8
  pour Top (isolate 0.254, no thermals): 18.48,22.67 10.35,22.67 6.16,26.86 4.38,26.86 4.32,26.92 4.32,27.24 4.38,27.3 4.64,27.3 5.27,27.94 6.98,27.94 10.79,24.13 18.54,24.13 18.67,24 18.67,22.86
N$10
  Top 0.406: C1.1 R3.2 R4.2
N$12
  Top 0.406: R5.2 R6.2 C3.1
P0
  Bottom 0.508: J3.1 LINKIT7688.1
P1  (via drill 0.3)
  Top 0.152: v62.36,31.88 62.36,36.45 J3.2 | EPHY.- v22.35,31.24
  Bottom 0.152: v62.36,31.88 22.99,31.88 v22.35,31.24
  Bottom 0.508: J3.2 LINKIT7688.2
P2/MDI_P0_RP  (via drill 0.3)
  Top 0.152: R5.1 20.07,41.15 v19.81,41.4 19.56,41.66 J7.P4
  Bottom 0.152: LINKIT7688.3 J3.3 73.15,44.7 65.02,44.7 63.12,46.61 21.08,46.61 18.54,44.07 18.54,42.04 18.92,41.66 19.56,41.66 v19.81,41.4
P3/MDI_P0_RN  (via drill 0.3)
  Top 0.152: R6.1 20.19,42.67 v19.81,42.29 19.18,42.93 J7.P5
  Bottom 0.152: LINKIT7688.4 J3.4 73.03,44.32 64.9,44.32 62.99,46.23 21.34,46.23 18.92,43.81 18.92,42.29 19.18,42.04 19.56,42.04 v19.81,42.29
P4/MDI_P0_TP  (via drill 0.3)
  Top 0.152: R3.1 20.19,38.1 v19.81,38.48 19.18,39.12 J7.P2
  Bottom 0.152: LINKIT7688.5 J3.5 73.91,40.64 73.03,39.75 67.95,39.75 62.36,45.34 23.37,45.34 21.97,43.94 21.97,41.4 20.45,39.88 19.43,39.88 19.18,39.62 19.18,39.12 v19.81,38.48
P5/MDI_P0_TN  (via drill 0.3)
  Top 0.152: R4.1 20.19,39.62 v19.81,39.24 19.81,39.88 19.3,40.39 J7.P3
  Bottom 0.152: LINKIT7688.6 J3.6 73.91,38.1 72.64,39.37 67.82,39.37 62.23,44.96 23.62,44.96 22.35,43.69 22.35,41.15 20.45,39.24 v19.81,39.24
P6/USB_DP  (via drill 0.3)
  Top 0.152: R2.2 20.19,10.67 22.86,10.67 23.88,11.68 23.88,22.35 24.45,22.92 24.51,22.99 24.64,23.11 24.64,33.4 v24.89,33.66
  Bottom 0.152: LINKIT7688.7 J3.7 74.17,35.43 72.26,33.53 25.02,33.53 v24.89,33.66
P7/USB_DN  (via drill 0.3)
  Top 0.152: R1.2 20.07,11.05 22.73,11.05 23.49,11.81 23.49,22.48 24.26,23.24 24.26,33.4 v24,33.66
  Bottom 0.152: LINKIT7688.8 J3.8 24.64,33.02 v24,33.66
P8/UART_TX2  (via drill 0.3)
  Top 0.152: v89.54,18.41 77.47,30.48 LINKIT7688.9
  Bottom 0.152: LINKIT7688.9 J3.9 | J4.2 v89.54,18.41
P9/UART_RX2  (via drill 0.3)
  Top 0.152: LINKIT7688.10 78.74,27.94 90.81,15.88 v92.08,15.88
  Bottom 0.152: LINKIT7688.10 J3.10 | J4.1 v92.08,15.88
RESET  (via drill 0.3)
  Top 0.152: v18.16,5.33 K1.1 | U2.36 64.14,12.45 v64.26,12.32
  Top 0.203: RST.- 17.65,3.17 K1.1
  Bottom 0.152: J2.19 LINKIT7688.39 83.95,5.08 78.74,10.29 78.74,15.11 77.47,16.38 72.39,16.38 69.85,13.84 65.79,13.84 v64.26,12.32 59.18,7.24 54.74,7.24 51.56,4.06 35.18,4.06 U2.30 30.73,5.46 24.51,5.46 RESET.T 23.37,4.32 19.3,4.32 18.29,5.33 v18.16,5.33
S0/MISO
  Top 0.152: J2.1 LINKIT7688.21 98.43,50.8 95.12,47.5 95.12,39.75 92.08,36.7 73.03,36.7 68.07,31.75 65.41,31.75 U2.38
S1/MOSI
  Top 0.152: J2.2 LINKIT7688.22 95.76,44.26 95.76,39.75 92.2,36.2 79.38,36.2 77.47,34.29 73.53,34.29 67.18,27.94 U2.34
S2/SCK
  Top 0.152: J2.3 LINKIT7688.23 99.63,45.59 98.04,45.59 96.52,44.07 96.52,39.88 92.33,35.69 81.66,35.69 77.72,31.75 73.15,31.75 68.07,26.67 65.79,26.67 64.52,27.94 U2.37
S3/SS
  Top 0.406: LINKIT7688.24 J2.4
UART_RX
  Bottom 0.152: J2.5 LINKIT7688.25 88.2,52.2 72.9,52.2 71.5,50.8 U2.1
UART_TX
  Bottom 0.152: J2.6 LINKIT7688.26 88.33,49.53 72.77,49.53 72.64,49.4 62.99,49.4 U2.2
USB_5V  (via drill 0.3, 0.36)
  Top 0.406: v24.64,9.27 24.77,9.27 25.27,9.78 25.27,20.07 v25.53,20.32
  Top 0.813: U2.28 38.73,7.49 39.62,8.38 v39.62,18.54 | LINKIT7688.14 C8.2 v81.28,17.78
  Bottom 0.406: USB5V.T 23.49,8.13 v24.64,9.27
  Bottom 0.813: LINKIT7688.14 J3.14 | J4.3 87,12.06 v81.28,17.78
  Bottom 1.016: 39.88,18.29 v39.62,18.54 | v39.62,18.54 29.84,18.54 27.94,20.32 v25.53,20.32 22.86,20.32 v21.21,18.67 | J3.14 40.39,17.78 v39.62,18.54
  other vias: 21.59,19.3
  pour Top (isolate 0.254, no thermals): 16.64,18.03 21.72,18.03 21.97,18.29 21.97,20.83 21.72,21.08 16.64,21.08 16.51,20.95 16.51,18.16

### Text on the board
tPlace: Ethernet | P0 | S0 | P1 | S1 | TX | RX | P2 | S2 | P3 | S3 | P4 | D0 | P5 | D1 | P6 | D2 | ICSP | P7 | D3 | P8 | D4 | PWR | P9 | D5 | ~ | GND | D6 | ~ | 3V3 | D7 | VIN | D8 | 5V | D9 | ~ | A0 | D10 | GND | 5V | TX2 | RX2 | ~ | A1 | D11 | I2C | I2C | I2C | ~ | A2 | D12 | A3 | D13 | Debug | ~ | RESET | A4 | RST | A5 | AREF
bPlace: PORST | S0/PB3 | 13 | 12 | 11 | 10 | 9 | 8 | 7 | 6 | 5 | 4 | 3 | 2 | 1 | 0 | SCL | SDA | ~ | ~ | ~ | ~ | ~ | ~ | JTDO | S1/PB2 | AREF | TX | RX | MDI_RP | S2/PB1 | GND | GND | GND | GND | MDI_RN | S3/PB0 | 3V3 | 3V3 | 3V3 | 3V3 | MDI_TP | D0/PD2 | A1 | A2 | A3 | D5 | MDI_TN | D1/PD3 | A0 | A1 | A2 | D4 | USB_DP | D2/PD1 | USB_DM | D3/PD0 | TXD2 | D4/PD4 | GND | GND | GND | GND | D5/PC6 | 3V3 | 3V3 | 3V3 | 3V3 | RXD2 | D6 | D7 | D8 | D9 | D6/PD7 | D5 | D6 | D7 | D8 | MISO | 3V3 | SCK | MOSI | D7/PE6 | RST | GND | D8/PB4 | D9/PB5 | GND | GND | GND | GND | A0/PF0 | D10/PB6 | 3V3 | 3V3 | 3V3 | 3V3 | A1/PF1 | www.seeedstudio.com | by Seeed Studio | v1.1 11/09/2015 | Arduino Breakout for LinkIt Smart 7688 Duo | D11/PB7 | SDA | SDA | SDA | D10 | A2/PF4 | D12/PD6 | SCL | SCL | SCL | D9 | GND | 5V | TX2 | RX2 | A3/PF5 | D13/PC7 | Debug | RESET | NC | IOREF | RST | 3V3 | 5V | NC | 0 | 1 | 2 | 3 | 4 | 5 | A4/PF6 | A5/PF7 | AREF | RST
Reference: HOST

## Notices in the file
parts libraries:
moudle-new: This work is licensed under the Creative Commons Attribution 4.0 International License.
To view a copy of this license,visit:
http://creativecommons.org/licenses/by-sa/4.0
moudle-new: CC-BY-SA
